// TwinCAT 3 PLC project Untitled1
// ProgramVersion: 3.1.4024.0
// libraries:
//   Tc2_Standard, * (Beckhoff Automation GmbH)
//   Tc2_System, * (Beckhoff Automation GmbH)
//   Tc3_Module, * (Beckhoff Automation GmbH)
// project tree:
//   / PlcTask.TcTTO
//   POUs/ MAIN.TcPOU
// real-time tasks:
//   TASK PlcTask: cycle T#1ms, priority 20, ADS port 350
// I/O:
//   DEVICE Gerät 2 (EtherCAT), AmsNetId 192.168.56.129.3.1
//     Klemme 1 (EK1101) [EK1101 EtherCAT-Koppler (2A E-Bus, ID-Switch)]
//       Klemme 2 (EL7041) [EL7041 1K. Schrittmotor-Endstufe (50V, 5A)]
//       Klemme 3 (EL7041) [EL7041 1K. Schrittmotor-Endstufe (50V, 5A)]
//       Klemme 4 (EL7041) [EL7041 1K. Schrittmotor-Endstufe (50V, 5A)]
//       Klemme 5 (EL1008) [EL1008 8K. Dig. Eingang 24V, 3ms]
//       Klemme 6 (EL6731) [EL6731 PROFIBUS DP Master]
//       Klemme 7 (EL9011) [EL9011 Endklemme]
//   DEVICE Gerät 1 (EL6731), AmsNetId 192.168.56.129.2.1
//     Box 10  (BK3150) // Buskoppler, 12MBaud Vendor: BECKHOFF Revision: Revision 4.03
//     Box 9 (GSD Box) (SINUMERIK MPP) // Vendor: SIEMENS Revision: V1.0
// variable links:
//   Untitled1/Untitled1 Instance <-> Device 1 (EL6731)
//     PlcTask Inputs/MAIN.inputEL <-> Inputs/ActualModulo
//   Untitled1/Untitled1 Instance <-> Device 1 (EL6731)/Box 10  (BK3150)
//     PlcTask Inputs/MAIN.boolTEST <-> Term 2 (KL1408)/Channel 1/Eingang
//     PlcTask Inputs/MAIN.dpState1 <-> Inputs/DpState
//     PlcTask Outputs/MAIN.bool2TEST <-> Term 4 (KL2408)/Channel 1/Ausgang
//   Untitled1/Untitled1 Instance <-> Device 1 (EL6731)/Box 9 (GSD Box) (SINUMERIK MPP)
//     PlcTask Inputs/MAIN.dpState2 <-> Inputs/DpState

CONFIGURATION Untitled1
    RESOURCE PLC ON TwinCAT3
        TASK PlcTask(INTERVAL := T#1ms, PRIORITY := 20);
        PROGRAM MAIN WITH PlcTask : MAIN;
    END_RESOURCE
END_CONFIGURATION

// ---- POUs/MAIN.TcPOU
PROGRAM MAIN
VAR
	inputEL AT %I*:INT;
	dpState1 AT %I* :USINT;
	dpState2 AT %I* :USINT;
	boolTEST AT %I* :BOOL;
	bool2TEST AT %Q* :BOOL;
END_VAR

END_PROGRAM
